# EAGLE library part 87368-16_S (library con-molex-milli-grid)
RECEPTACAL
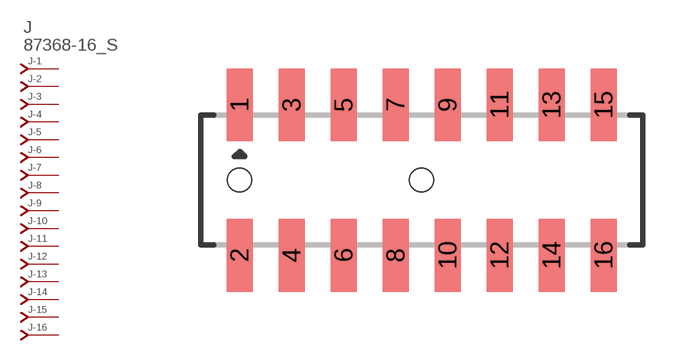
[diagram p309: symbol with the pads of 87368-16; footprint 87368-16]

Designator prefix J; gates -1=J-NV -2=J-N -3=J-N -4=J-N -5=J-N -6=J-N -7=J-N -8=J-N -9=J-N -10=J-N -11=J-N -12=J-N -13=J-N -14=J-N -15=J-N -16=J-N

## 87368-16_S  [87368-16]
1  -1:J  pas
2  -2:J  pas
3  -3:J  pas
4  -4:J  pas
5  -5:J  pas
6  -6:J  pas
7  -7:J  pas
8  -8:J  pas
9  -9:J  pas
10  -10:J  pas
11  -11:J  pas
12  -12:J  pas
13  -13:J  pas
14  -14:J  pas
15  -15:J  pas
16  -16:J  pas

## Footprint 87368-16 (pad centres in mm)
RECEPTACAL SMD Dual Row, Side Entry
smd 1 x 2.8: 1 -7,2.9; 2 -7,-2.9; 3 -5,2.9; 4 -5,-2.9; 5 -3,2.9; 6 -3,-2.9; 7 -1,2.9; 8 -1,-2.9; 9 1,2.9; 10 1,-2.9; 11 3,2.9; 12 3,-2.9; 13 5,2.9; 14 5,-2.9; 15 7,2.9; 16 7,-2.9
hole 0.914 at -7,0
hole 0.914 at 0,0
